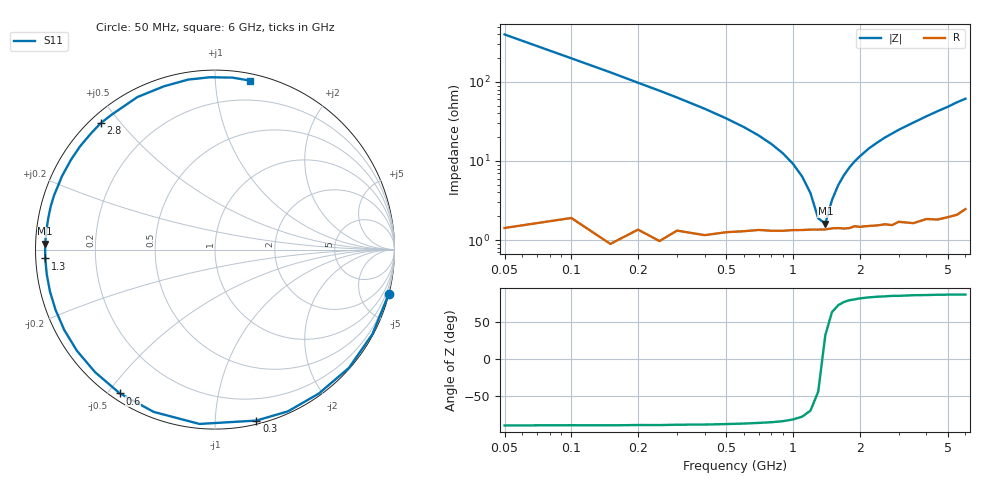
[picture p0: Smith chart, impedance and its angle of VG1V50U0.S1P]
! Infineon Technologies  Discrete & RF Semiconductors
! BB 831
! Si Tuning Diode in SOD323
! VR = 1.5 V
! S-Parameters:  July  1999
# GHz  S  MA  R  50
!  f  S11
! GHz  MAG  ANG
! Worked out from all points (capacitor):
!   34 points, 50 MHz to 6 GHz, reference 50 ohm
!   read as one part to ground: C = 7.95 pF near 50 MHz
!   lowest |Z| = 1.62 ohm at 1.4 GHz (marker M1)
!   series resonance near 1.36 GHz, so ESL is about 1.7 nH
!   S11 on the Smith chart (normalised r, x): 50 MHz: 0.03, -7.97; 300 MHz: 0.03, -1.27; 600 MHz: 0.03, -0.54; 1.3 GHz: 0.03, -0.03; 2.8 GHz: 0.03, +0.44; 6 GHz: 0.05, +1.22
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0.05  0.9991 -14.3
0.1  0.9955 -28.2
0.15  0.9956 -41.4
0.2  0.9888 -54.2
0.25  0.9886 -65.7
0.3  0.9801 -76.4
0.4  0.9752 -95.1
0.5  0.9666 -110.7
0.6  0.9607 -123.5
0.7  0.9554 -134.4
0.8  0.9537 -143.8
0.9  0.9519 -152.0
1  0.9496 -159.3
1.1  0.9487 -165.8
1.3  0.9473 -177.0
1.4  0.947 178.0
1.6  0.9454 169.2
1.8  0.9463 161.4
2  0.9456 154.5
2.2  0.9458 148.0
2.4  0.9467 142.4
2.8  0.9497 132.1
3.5  0.9536 117.0
4  0.9532 107.4
4.5  0.9589 99.0
5  0.9607 91.7
5.5  0.9631 84.2
6  0.9614 78.4
